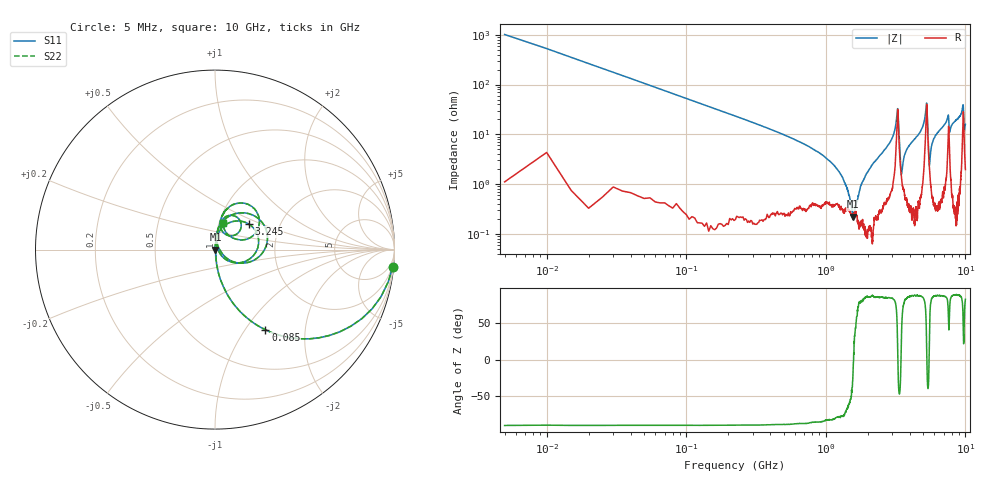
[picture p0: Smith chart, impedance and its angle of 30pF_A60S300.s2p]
! Amotech Co.,Ltd.
! http://www.amotech.co.kr/
! Part Number: A60S300
! These Parameters are Measured in Series Mode Connection
! Operation Temp=25[degC], DC Bias Voltage=0[V]
! Freq. Start=5[MHz] Stop=10[GHz], 2000[Steps]
! Date: Monday, July 13, 2020, 01:40:32
# GHZ S RI R 50.000000
!Freq.(Hz) S11(Real) S11(Imag) S21(Real) S21(Imag) S12(Real) S12(Imag) S22(Real) S22(Imag)
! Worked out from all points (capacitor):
!   2000 points, 5 MHz to 10 GHz, reference 50 ohm
!   read as one part in series: C = 30 pF near 55 MHz
!   lowest |Z| = 220 mohm at 1.575 GHz (marker M1)
!   series resonance near 1.581 GHz, so ESL is about 340 pH
!   S11 on the Smith chart (normalised r, x): 5 MHz: 1, -20; 85 MHz: 1.01, -1.25; 3.245 GHz: 1.39, +0.42; 10 GHz: 1.04, +0.32
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0.005  0.9903 -0.0974  0.00968 0.0974  0.00968 0.0974  0.9903 -0.0974
0.085  0.2808 -0.4461  0.7192 0.4461  0.7192 0.4461  0.2808 -0.4461
0.275  0.036 -0.1819  0.964 0.1819  0.964 0.1819  0.036 -0.1819
1.27  0.00326 -0.0157  0.9967 0.0157  0.9967 0.0157  0.00326 -0.0157
1.575  0.00219 -0.000187  0.9978 0.000187  0.9978 0.000187  0.00219 -0.000187
1.675  0.00235 0.00405  0.9976 -0.00405  0.9976 -0.00405  0.00235 0.00405
1.965  0.00117 0.0166  0.9988 -0.0166  0.9988 -0.0166  0.00117 0.0166
2.975  0.014 0.0795  0.986 -0.0795  0.986 -0.0795  0.014 0.0795
3.245  0.1877 0.1426  0.8123 -0.1426  0.8123 -0.1426  0.1877 0.1426
3.34  0.0794 -0.0653  0.9206 0.0653  0.9206 0.0653  0.0794 -0.0653
3.49  0.0124 0.0095  0.9876 -0.0095  0.9876 -0.0095  0.0124 0.0095
3.825  0.00685 0.0506  0.9932 -0.0506  0.9932 -0.0506  0.00685 0.0506
5.005  0.0375 0.149  0.9625 -0.149  0.9625 -0.149  0.0375 0.149
5.28  0.292 0.054  0.708 -0.054  0.708 -0.054  0.292 0.054
5.53  0.0194 0.0135  0.9806 -0.0135  0.9806 -0.0135  0.0194 0.0135
5.89  0.0103 0.0767  0.9897 -0.0767  0.9897 -0.0767  0.0103 0.0767
6.67  0.0206 0.1247  0.9794 -0.1247  0.9794 -0.1247  0.0206 0.1247
7.7  0.0507 0.0906  0.9493 -0.0906  0.9493 -0.0906  0.0507 0.0906
8.335  0.0334 0.1726  0.9666 -0.1726  0.9666 -0.1726  0.0334 0.1726
9.59  0.2027 0.2421  0.7973 -0.2421  0.7973 -0.2421  0.2027 0.2421
9.805  0.0776 0.0791  0.9224 -0.0791  0.9224 -0.0791  0.0776 0.0791
10  0.0425 0.1495  0.9575 -0.1495  0.9575 -0.1495  0.0425 0.1495
